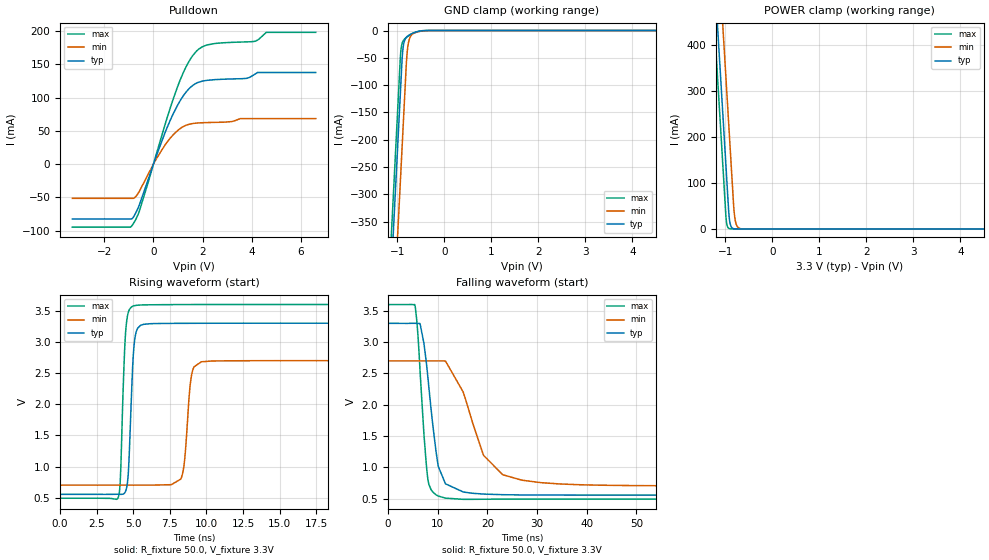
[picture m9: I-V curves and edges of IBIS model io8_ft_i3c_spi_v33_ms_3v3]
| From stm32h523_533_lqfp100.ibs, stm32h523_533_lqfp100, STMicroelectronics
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[Model]   io8_ft_i3c_spi_v33_ms_3v3
Model_type I/O_open_drain
Polarity   Non-Inverting
Enable   Active-Low
| CAP_THRESHOLD on pad IOFT is "UDTCAPC" :
| Rising=20.0% of vddiom   Falling=80.0% of vddiom
| C_comp min and max val. don't necessarily correlate with the min and max pvt
| but are the smallest and greatest pad capacitance found.
| var   typ   min   max
C_comp   3.95302pF  3.95027pF  4.00767pF
|C_comp_pulldown   3.95302pF  3.95027pF  4.00767pF
Vinl = 1.35V
Vinh = 1.8V
Vmeas = 1.65V   | Reference voltage for timing measurements
Cref  = 50.0pF   | Timing specification test load capacitance value
Rref  = 1.0MOhm   | Timing specification test load resistance value
Vref  = 1.815V   | Timing specification test load voltage
[Model Spec]
| TIME_THRESHOLD on pin ZII2CV11 is "CMOS" :
| Rising=40.0% of vdd   Falling=60.0% of vdd
Vinl 1.28680V 1.06380V 1.39380V
Vinh 1.76920V 1.48820V 1.89120V
| variable   typ   min   max
[Temperature Range] 25.0 125.0 -40.0
| variable   typ   min   max
[Voltage Range] 3.3V 2.7V 3.6V
| variable   typ   min   max
[POWER Clamp Reference] 3.3V 2.7V 3.6V
| variable   typ   min   max
[GND Clamp Reference] 0V 0V 0V
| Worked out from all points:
|   slope of the pulldown table from 0 to 0.495 V, typ, clamps not added: 10 ohm
|   GND clamp passes 1 mA (typ) near -0.52 V on its own axis
|   POWER clamp passes 1 mA (typ) near -0.84 V on its own axis
|   rising waveform, R_fixture 50.0, V_fixture 3.3V: 20-80 % time 285ps typ, 379ps min, 266ps max; typ from 0.556 V to 3.3 V
|   falling waveform, R_fixture 50.0, V_fixture 3.3V: 20-80 % time 2.35ns typ, 5.9ns min, 1.5ns max; typ from 3.3 V to 0.556 V
[POWER Clamp]
-3.3V     4.068A     4.259A     3.957A
-1.25V    582.8mA    774.2mA    471.5mA
-1.21V    514.8mA    706.2mA    403.5mA
-1.13V    378.8mA    570.2mA    267.5mA
-1.04V    225.8mA    417.2mA    114.5mA
-980mV    123.8mA    315.2mA    17.95mA
-920mV    26.3mA     213.2mA    906uA
-880mV    5.543mA    145.2mA    123.7uA
-810mV    363.5uA    33.6mA     3.798uA
-770mV    76.62uA    10.47mA    519.4nA
-690mV    3.409uA    1.017mA    10.47nA
6.6V      0A         0A         0A
[GND Clamp]
-3.3V     -4.13A     -4.291A    -4.063A
-1.25V    -644.7mA   -806.4mA   -578.1mA
-940mV    -117.7mA   -279.4mA   -51.06mA
-920mV    -83.75mA   -245.4mA   -31.43mA
-900mV    -50.5mA    -211.4mA   -23.14mA
-880mV    -31.27mA   -177.4mA   -19.1mA
-850mV    -18.68mA   -126.4mA   -15.73mA
-800mV    -11.46mA   -46.4mA    -12.03mA
-760mV    -8.752mA   -20.02mA   -9.606mA
-680mV    -5.122mA   -6.673mA   -5.579mA
-300mV    -5.379uA   -47.63uA   -852.7nA
6.6V      10.49nA    1.843uA    393.6pA
| variable   typ   min   max
[Pullup Reference] 3.3V 2.7V 3.6V
| variable   typ   min   max
[Pulldown Reference] 0V 0V 0V
[Pulldown]
-3.3V     -82.42mA   -51.49mA   -94.82mA
-850mV    -81.27mA   -51.49mA   -91.26mA
-580mV    -62.01mA   -41.36mA   -71.41mA
120mV     12.61mA    7.999mA    15.37mA
800mV     75.3mA     43.94mA    97.52mA
1.33V     108.3mA    58.37mA    146.5mA
1.84V     123.1mA    61.83mA    172.7mA
2.51V     126.9mA    62.7mA     181.3mA
3.78V     128.8mA    68.32mA    183.7mA
4.12V     134.9mA    68.32mA    184.6mA
4.59V     137.6mA    68.32mA    198mA
6.6V      137.6mA    68.32mA    198mA
[Ramp]
dV/dt_r 1.64663V/282.76822ps 1.19796V/377.51866ps 1.86385V/262.64365ps
dV/dt_f 1.64666V/2.32519ns 1.19801V/5.11622ns 1.86387V/1.50254ns
R_load = 50.0
| Removed startup time: 0s 0s 0s  .
| Removed end time: 33.7ns.
[Rising Waveform]
R_fixture   = 50.0
V_fixture   = 3.3V
V_fixture_min = 2.7V
V_fixture_max = 3.6V
0s        555.6mV    703.3mV    493.6mV
3.95ns    557.7mV    703.3mV    494.3mV
4.1ns     556.6mV    703.3mV    725.6mV
4.4ns     575mV      703.3mV    2.841V
4.6ns     740.8mV    703.3mV    3.416V
5ns       2.796V     703.3mV    3.576V
8.25ns    3.298V     802mV      3.599V
8.95ns    3.298V     2.424V     3.599V
9.65ns    3.299V     2.681V     3.6V
33.7ns    3.3V       2.7V       3.6V
| Removed startup time: 0s 0s 0s  .
| Removed end time: 188.7ns.
[Falling Waveform]
R_fixture   = 50.0
V_fixture   = 3.3V
V_fixture_min = 2.7V
V_fixture_max = 3.6V
0s        3.3V       2.7V       3.6V
5.4ns     3.301V     2.7V       3.595V
6.5ns     3.272V     2.7V       2.455V
8.05ns    2.41V      2.7V       793.4mV
10.1ns    1.016V     2.7V       541.2mV
11.55ns   736.7mV    2.699V     507.4mV
15.1ns    607.5mV    2.207V     488.8mV
19.25ns   572.3mV    1.188V     490mV
26.95ns   558.6mV    794.2mV    492.9mV
188.7ns   555.6mV    703.3mV    493.6mV
